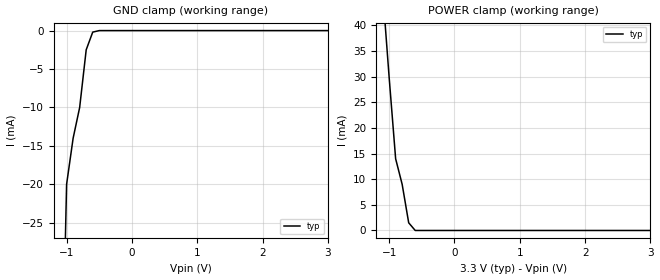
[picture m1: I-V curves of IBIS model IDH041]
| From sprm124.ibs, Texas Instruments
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|****** ****   ***** *****   ******  Buffer Models  ***************************
[Model]   IDH041
Model_type   Input
Polarity   Non-Inverting
| signals
Vinl = 0.8V
Vinh = 2.0V
|   typ   min   max
C_comp   1.9230p   1.9076p   2.1739p
|   typ   min   max
[Temperature Range]   25.0   0   90
|   typ   min   max
[Voltage Range]   3.3V   3.13V   3.47V
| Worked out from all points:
|   GND clamp passes 1 mA (typ) near -0.63 V on its own axis
|   POWER clamp passes 1 mA (typ) near -0.67 V on its own axis
[GND_clamp]
|   Voltage   I(typ)   I(min)   I(max)
-3V       -900mA     NA         NA
-2V       -400mA     NA         NA
-1V       -20mA      NA         NA
-900mV    -14mA      NA         NA
-800mV    -10mA      NA         NA
-700mV    -2.5mA     NA         NA
-600mV    -200uA     NA         NA
-500mV    0A         NA         NA
3V        0A         NA         NA
[POWER_clamp]
|   Voltage   I(typ)   I(min)   I(max)
-3V       600mA      NA         NA
-2V       200mA      NA         NA
-1V       30mA       NA         NA
-900mV    14mA       NA         NA
-800mV    9mA        NA         NA
-700mV    1.5mA      NA         NA
-600mV    0A         NA         NA
-500mV    0A         NA         NA
3V        0A         NA         NA
